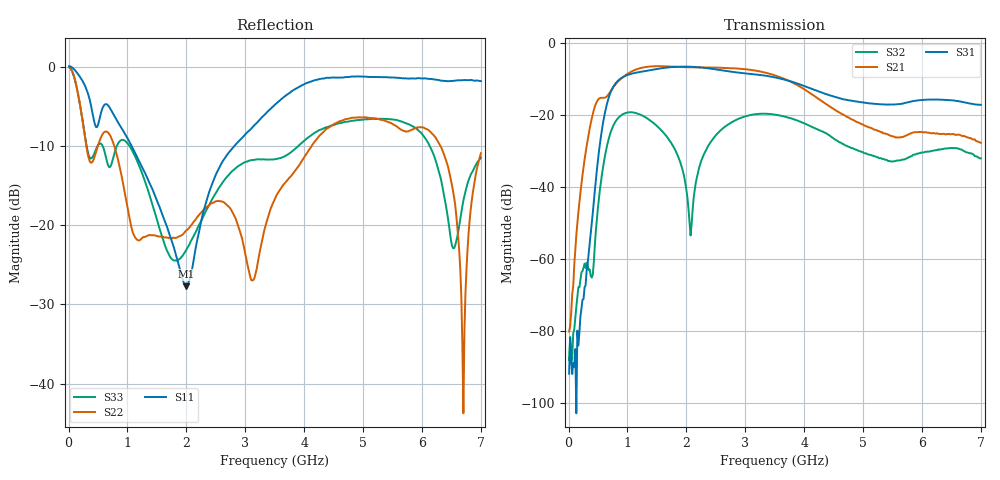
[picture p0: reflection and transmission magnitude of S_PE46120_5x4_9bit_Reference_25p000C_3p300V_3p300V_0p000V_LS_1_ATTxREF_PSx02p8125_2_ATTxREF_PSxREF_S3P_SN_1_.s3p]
! Device ID: PE46120_5x4_9bit_Reference
! Device ID: PE46120_5x4_9bit_Reference
! File Path: z:\PE46120_5x4_9bit_Reference\MPAC_Yi\new_12port\25p000C\3p300\LS_1_ATTxREF_PSx02p8125_2_ATTxREF_PSxREF\PE46120_5x4_9bit_Reference_25p000C_3p300V_3p300V_0p000V_LS_1_ATTxREF_PSx02p8125_2_ATTxREF_PSxREF_S3P_SN_1_.s3p
! Serial: 1
! Lot:
! Temp: 25.000C
! VDD: 3.300
! VSS: 0.000
! Control_Hi: 3.300
! Control_Lo: 0.000
! Logic State: LS_1_ATTxREF_PSx02p8125_2_ATTxREF_PSxREF
! Port 1: RFin
! Port 2: RFout1
! Port 3: RFout2
! ThroughPath:1-2
! IDD: -0.0005430565
! ISS: 0
! Comment:
#  Hz  S  RI  R  50
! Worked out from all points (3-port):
!   401 points, 10 MHz to 7 GHz, reference 50 ohm
!   strongest paths, dB at 10 MHz, 1.758 GHz, 3.505 GHz, 5.253 GHz, 7 GHz:
!     S31: -91.7, -6.7, -9.5, -16.9, -17.1
!     S21: -80.1, -6.5, -9.0, -24.4, -27.7
!     S32: -87.9, -28.1, -19.9, -31.7, -32.0
!   lowest |S11| = -27.7 dB at 2.002 GHz (marker M1), VSWR 1.09, Z = 53.4 + j2.55 ohm
!   |S11| at or under -10 dB: 1.071 GHz to 2.815 GHz (1.745 GHz wide, 89.8 % of centre)
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1e7  1.002 -0.1147  0.00012 -1.56e-05  -9e-06 7.95e-05
     -7.93e-06 9.89e-05  0.9887 -0.0959  5.57e-05 -1.94e-05
     -1.31e-05 2.23e-05  -2.87e-05 -2.82e-05  0.9879 -0.0961
2.5465e8  -0.5317 -0.5875  -0.0177 -0.00579  0.000175 0.000248
          -0.018 -0.00592  -0.3196 -0.266  -0.000164 0.000617
          0.000122 0.000253  -0.000315 0.000694  -0.3249 -0.2626
4.81825e8  -0.4044 -0.0933  -0.0394 0.1474  0.0171 0.00301
           -0.0395 0.1493  0.2012 0.2251  -0.00242 0.00269
           0.0173 0.00296  -0.00234 0.0028  0.2073 0.2318
9.71125e8  -0.2588 0.2639  0.3342 -0.1208  -0.0571 0.3438
           0.3384 -0.1227  -0.078 -0.1264  -0.0277 0.1023
           -0.057 0.3477  -0.0276 0.1037  0.0742 -0.3296
2.00215e9  0.0336 0.0239  -0.3413 0.3034  -0.3041 -0.353
           -0.3452 0.3076  -0.0395 0.0842  0.00226 0.00829
           -0.3081 -0.3564  0.00256 0.00864  -0.0702 0.00423
2.806e9  -0.0858 -0.3015  0.4354 0.0723  -0.0975 0.3796
         0.4408 0.0723  0.0989 -0.0609  0.0168 0.0799
         -0.0974 0.3844  0.017 0.0809  0.0667 0.2132
3.505e9  -0.4279 -0.3867  -0.1141 -0.3321  0.3254 0.0536
         -0.1157 -0.3367  0.0873 0.1183  0.00345 -0.1006
         0.3296 0.0536  0.00318 -0.1017  0.1877 -0.1813
6.108775e9  -0.4399 0.7137  0.0464 -0.0312  -0.0615 0.1499
            0.0471 -0.032  0.3983 -0.0271  -0.0259 -0.0172
            -0.0622 0.152  -0.0259 -0.0172  0.3049 -0.1235
6.702925e9  -0.2323 0.7905  -0.0118 -0.0491  0.0991 0.1118
            -0.0129 -0.0498  -0.00642 -0.000941  0.0115 0.029
            0.1006 0.1127  0.0124 0.0295  0.0736 0.1228
7e9  -0.1164 0.8036  -0.0321 -0.0247  0.1247 0.0561
     -0.0329 -0.025  0.0166 0.284  0.024 -0.00166
     0.1272 0.0564  0.0251 -0.00166  0.1463 0.2222
